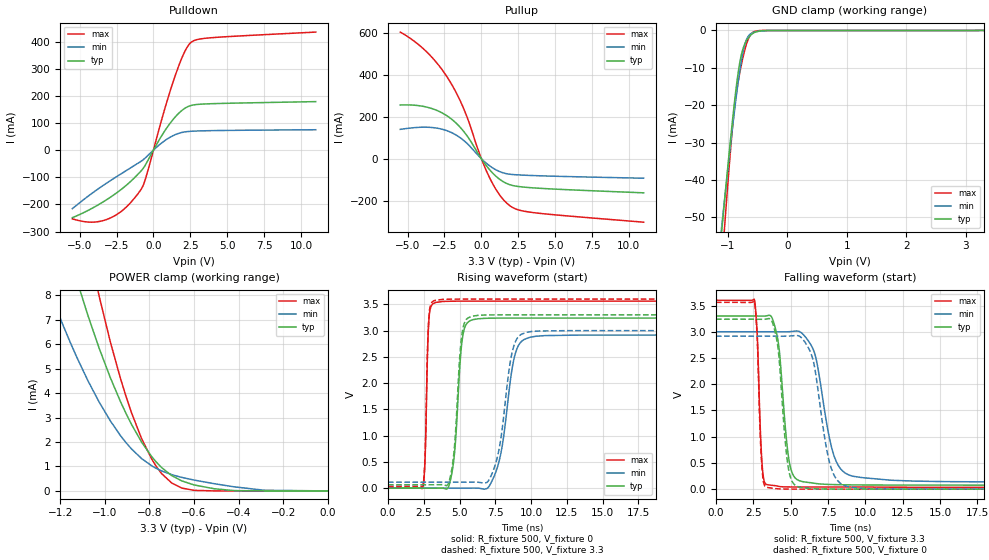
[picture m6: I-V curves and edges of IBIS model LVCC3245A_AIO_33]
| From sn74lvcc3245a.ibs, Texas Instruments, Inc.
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[Model]   LVCC3245A_AIO_33
Model_type  I/O
Vinl=0.8
Vinh=2.0
Enable   Active-Low
Vref =   0
Rref =   500
Cref =   50p
Vmeas =   1.5
| variable   typ   min   max
C_comp   18.50pF   NA   NA
| C_pullup   12.57pF   9.06pF   15.78pF
| C_pulldown   8.35pF   3.33pF   12.56pF
| C_tri-state   7.99pF   6.87pF   9.01pF
[Temperature Range]   40   100   -40
| Ambient temperature   25   85   -40
[Voltage range]   3.3   3   3.6
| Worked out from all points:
|   slope of the pulldown table from 0 to 0.495 V, typ, clamps not added: 10.5 ohm
|   slope of the pullup table from 0 to 0.495 V, typ, clamps not added: 10.5 ohm
|   GND clamp passes 1 mA (typ) near -0.60 V on its own axis
|   POWER clamp passes 1 mA (typ) near -0.75 V on its own axis
|   rising waveform, R_fixture 500, V_fixture 0: 20-80 % time 454ps typ, 886ps min, 186ps max; typ from 0 V to 3.24 V
|   falling waveform, R_fixture 500, V_fixture 3.3: 20-80 % time 573ps typ, 1.09ns min, 260ps max; typ from 3.3 V to 0.065 V
|   rising waveform, R_fixture 500, V_fixture 3.3: 20-80 % time 441ps typ, 833ps min, 182ps max; typ from 0.064 V to 3.3 V
|   falling waveform, R_fixture 500, V_fixture 0: 20-80 % time 539ps typ, 944ps min, 248ps max; typ from 3.24 V to 0 V
[GND Clamp]
| LVCC3245A_AIO_33
|   Voltage   I(typ)   I(min)   I(max)
-5.5V     -942.2mA   -838.7mA   -1.112A
-1.14V    -60.03mA   -57.96mA   -71.14mA
-1.095V   -52.27mA   -51.13mA   -61.19mA
-1.055V   -45.47mA   -45.12mA   -52.49mA
-925mV    -24.46mA   -26.38mA   -26.38mA
-855mV    -14.61mA   -17.16mA   -16.45mA
-785mV    -7.338mA   -9.244mA   -10.09mA
-725mV    -3.983mA   -4.327mA   -5.777mA
-665mV    -2.177mA   -1.736mA   -2.624mA
-585mV    -832.2uA   -608.3uA   -556.3uA
-330mV    -6.631uA   -44.07uA   -516.8nA
3.3V      1.597nA    37.51uA    29.73pA
[POWER Clamp]
| LVCC3245A_AIO_33
|   Voltage   I(typ)   I(min)   I(max)
-5.5V     377.9mA    260.8mA    635.5mA
-1.25V    12.75mA    8.244mA    18.97mA
-1.215V   11.52mA    7.41mA     16.99mA
-1.125V   8.607mA    5.457mA    12.34mA
-1.075V   7.156mA    4.496mA    10.04mA
-1.025V   5.828mA    3.629mA    7.952mA
-930mV    3.658mA    2.266mA    4.607mA
-835mV    1.996mA    1.323mA    2.138mA
-770mV    1.188mA    924uA      1.012mA
-700mV    627.1uA    664.4uA    322.5uA
-510mV    89.41uA    296.3uA    1.164uA
-95.1fV   1.597nA    9.868nA    34.26pA
[Pulldown]
| LVCC3245A_AIO_33
|   Voltage   I(typ)   I(min)   I(max)
-5.5V     -248.9mA   -215.9mA   -253.2mA
-4.18V    -214.9mA   -159.8mA   -265.6mA
-3.02V    -177.3mA   -116.1mA   -252.3mA
-1.92V    -133.2mA   -78.07mA   -213.8mA
-880mV    -79.07mA   -42.55mA   -147.8mA
-540mV    -54.04mA   -28.08mA   -105.7mA
695mV     64.77mA    31.95mA    138.6mA
1.46V     121.1mA    56.44mA    272.1mA
2.095V    152.7mA    66.76mA    360mA
2.575V    164.7mA    69.38mA    397.8mA
3.92V     170.9mA    71.65mA    413.9mA
11V       178.6mA    74.97mA    434.7mA
[Pullup]
| LVCC3245A_AIO_33
|   Voltage   I(typ)   I(min)   I(max)
-5.5V     256.6mA    140.1mA    604.8mA
-3.71V    246.5mA    150.4mA    510.4mA
-2.93V    228mA      144.9mA    449.6mA
-2.23V    199.9mA    130.8mA    380mA
-1.165V   127.4mA    85.22mA    233.2mA
-70mV     7.573mA    5.016mA    13.01mA
520mV     -49.47mA   -32.11mA   -85.6mA
1.195V    -95.97mA   -60.28mA   -168.9mA
1.87V     -122.8mA   -73.61mA   -221.3mA
2.475V    -132.5mA   -77.26mA   -243.7mA
3.485V    -139.2mA   -80.46mA   -257.1mA
11V       -163mA     -93.23mA   -303.3mA
[Ramp]
| LVCC3245A_AIO_33
| variable   typ   min   max
dV/dt_r   1.95/4.63E-10   1.76/8.97E-10   2.14/1.89E-10
dV/dt_f   1.95/5.80E-10   1.74/1.09E-09   2.15/2.69E-10
R_load = 500
[Rising Waveform]
| LVCC3245A_AIO_33
R_fixture =   500
C_fixture =   0
L_fixture =   0
V_fixture =   0
V_fixture_min = 0
V_fixture_max = 0
|   Time   V(typ)   V(min)   V(max)
0s        173.3pV    118.9nV    65.79pV
2.435ns   -392nV     151.8nV    7.135mV
2.855ns   -4.826uV   332.1nV    3.194V
3.33ns    -42.32uV   -376.6nV   3.536V
4.37ns    159.9mV    -7.507uV   3.558V
5.2ns     2.85V      -66.78uV   3.56V
5.95ns    3.209V     1.608mV    3.561V
7.54ns    3.237V     307.3mV    3.561V
9.92ns    3.238V     2.873V     3.561V
50ns      3.239V     2.916V     3.561V
[Falling Waveform]
| LVCC3245A_AIO_33
R_fixture =   500
C_fixture =   0
L_fixture =   0
V_fixture =   3.3
V_fixture_min = 3
V_fixture_max = 3.6
|   Time   V(typ)   V(min)   V(max)
0s        3.3V       3V         3.6V
2.58ns    3.3V       3V         3.606V
3.07ns    3.298V     3V         553.9mV
3.395ns   3.304V     3V         87.1mV
4.155ns   2.824V     2.999V     56.09mV
4.95ns    459.4mV    3.002V     42.31mV
5.725ns   148.9mV    2.981V     41.4mV
7.935ns   87.06mV    609.5mV    40.98mV
9.19ns    81.41mV    245.6mV    40.96mV
50ns      65.17mV    122.4mV    34.19mV
[Rising Waveform]
| LVCC3245A_AIO_33
R_fixture =   500
C_fixture =   0
L_fixture =   0
V_fixture =   3.3
V_fixture_min = 3
V_fixture_max = 3.6
|   Time   V(typ)   V(min)   V(max)
0s        64.38mV    113.3mV    34.19mV
2.435ns   64.38mV    113.3mV    41.13mV
2.85ns    64.38mV    113.3mV    3.24V
3.3ns     64.35mV    113.3mV    3.576V
4.36ns    222.2mV    113.3mV    3.598V
5.155ns   2.904V     113.3mV    3.6V
5.865ns   3.273V     114.4mV    3.6V
7.41ns    3.299V     372.6mV    3.6V
9.67ns    3.3V       2.966V     3.6V
50ns      3.3V       3V         3.6V
[Falling Waveform]
| LVCC3245A_AIO_33
R_fixture =   500
C_fixture =   0
L_fixture =   0
V_fixture =   0
V_fixture_min = 0
V_fixture_max = 0
|   Time   V(typ)   V(min)   V(max)
0s        3.239V     2.916V     3.561V
2.575ns   3.239V     2.916V     3.57V
3.06ns    3.237V     2.916V     489mV
3.39ns    3.243V     2.916V     36.05mV
4.14ns    2.721V     2.915V     7.46mV
4.88ns    347.6mV    2.917V     1.584mV
5.605ns   37.53mV    2.912V     851.5uV
7.7ns     2.492mV    413.9mV    100.2uV
8.865ns   1.232mV    46.86mV    59.97uV
50ns      37.36uV    149.7uV    938.4nV
